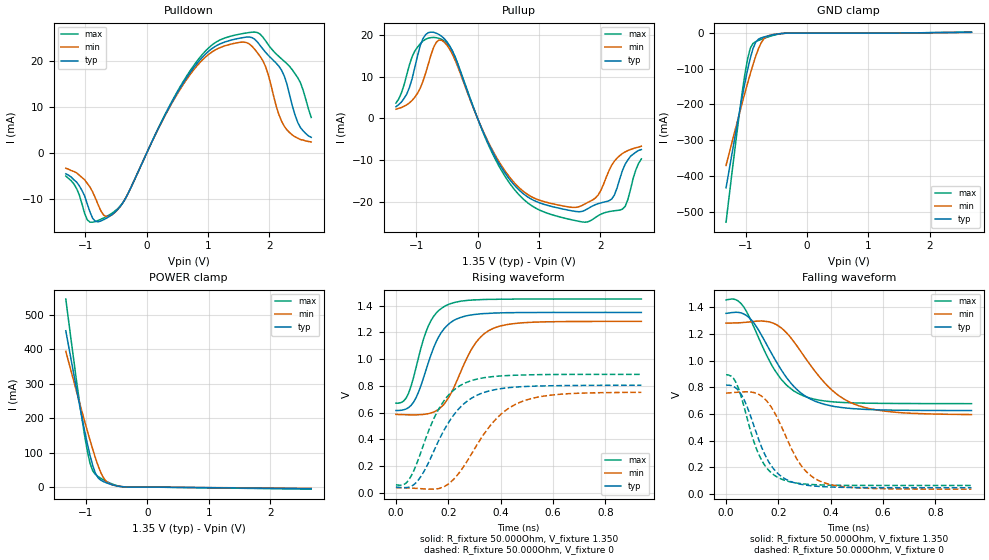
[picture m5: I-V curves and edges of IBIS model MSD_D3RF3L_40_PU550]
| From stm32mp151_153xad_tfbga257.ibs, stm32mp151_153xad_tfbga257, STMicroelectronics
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[Model] MSD_D3RF3L_40_PU550
Model_type   I/O
C_comp 2.425pF   2.340pF   2.550pF
Vinh = 810.000mV
Vinl = 540.000mV
Vmeas = 675.000mV
Vref = 675.000mV
[Model Spec]
Vinh   810.000mV   777.000mV   860.000mV
Vinl   540.000mV   507.000mV   590.000mV
Vmeas   675.000mV   642.000mV   725.000mV
Vref   675.000mV   642.000mV   725.000mV
[Temperature Range]   25.000   125.000   -40.000
[Voltage Range]   1.350V   1.283V   1.450V
[GND Clamp Reference]   0.00V   0.00V   0.00V
[Pulldown Reference]   0.00V   0.00V   0.00V
[POWER Clamp Reference]   1.350V   1.283V   1.450V
[Pullup Reference]   1.350V   1.283V   1.450V
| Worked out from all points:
|   slope of the pulldown table from 0 to 0.203 V, typ, clamps not added: 35.7 ohm
|   slope of the pullup table from 0 to 0.203 V, typ, clamps not added: 29.7 ohm
|   GND clamp passes 1 mA (typ) near -0.40 V on its own axis
|   POWER clamp passes 1 mA (typ) near -0.41 V on its own axis
|   rising waveform, R_fixture 50.000Ohm, V_fixture 1.350: 20-80 % time 86.8ps typ, 109ps min, 73.7ps max; typ from 0.615 V to 1.35 V
|   rising waveform, R_fixture 50.000Ohm, V_fixture 0: 20-80 % time 135ps typ, 161ps min, 116ps max; typ from 0.042 V to 0.804 V
|   falling waveform, R_fixture 50.000Ohm, V_fixture 1.350: 20-80 % time 147ps typ, 176ps min, 128ps max; typ from 1.35 V to 0.626 V
|   falling waveform, R_fixture 50.000Ohm, V_fixture 0: 20-80 % time 98.2ps typ, 116ps min, 84.8ps max; typ from 0.817 V to 0.048 V
[GND Clamp]
-1.318V   -433.6mA   -370.9mA   -529.9mA
-1.142V   -261.3mA   -253.2mA   -281mA
-1.055V   -178.7mA   -195.7mA   -165.9mA
-1.011V   -139.6mA   -167.6mA   -114.8mA
-966.7mV  -102.8mA   -140.1mA   -71.88mA
-922.7mV  -69.94mA   -113.6mA   -42.23mA
-878.8mV  -43.31mA   -88.24mA   -28.81mA
-790.9mV  -17.16mA   -44.13mA   -20.63mA
-703mV    -11.02mA   -16.16mA   -14.93mA
-527.3mV  -3.992mA   -3.373mA   -5.331mA
-307.6mV  -127.2uA   -185uA     -115.4uA
2.68V     2.404mA    2.042mA    2.844mA
[Power Clamp]
-1.33V    453mA      393.5mA    545mA
-1.111V   242.5mA    247.8mA    251.5mA
-1.023V   162.8mA    190.8mA    148.6mA
-978.8mV  125.6mA    162.8mA    104.1mA
-934.9mV  91.53mA    135.6mA    68.58mA
-890.9mV  62.14mA    109.2mA    46.94mA
-847mV    39.8mA     84.23mA    36.44mA
-803mV    26.44mA    61.41mA    30.34mA
-715.1mV  15.75mA    26.63mA    20.83mA
-671.2mV  12.52mA    16.53mA    16.67mA
-407.6mV  924.4uA    1.209mA    1.119mA
2.668V    -4.735mA   -3.8mA     -6.092mA
[Pulldown]
-1.318V   -4.5mA     -3.3mA     -5mA
-922.7mV  -12.81mA   -7.4mA     -14.98mA
-703mV    -14.45mA   -13.42mA   -14.07mA
-571.2mV  -13.38mA   -13.44mA   -13.08mA
-351.5mV  -9.986mA   -9.957mA   -9.952mA
747mV     18.14mA    17.69mA    18.58mA
1.098V    22.94mA    22.18mA    23.74mA
1.582V    25.02mA    24.02mA    25.91mA
1.889V    22.57mA    20.05mA    25.16mA
2.241V    16.68mA    5.8mA      19.86mA
2.461V    6.6mA      3.2mA      16.3mA
2.68V     3.4mA      2.4mA      7.7mA
[Pullup]
-1.33V    2.8mA      2.205mA    3.679mA
-1.155V   5.8mA      3.257mA    10.41mA
-978.8mV  15mA       6.025mA    17.12mA
-715.1mV  20.69mA    17.11mA    19.47mA
-451.5mV  17.37mA    16.56mA    17.25mA
251.5mV   -8.249mA   -7.87mA    -8.718mA
866.7mV   -19.34mA   -18.75mA   -20.84mA
1.702V    -22.37mA   -20.93mA   -24.89mA
1.965V    -20.5mA    -18.41mA   -23.39mA
2.185V    -19.39mA   -11.26mA   -22.3mA
2.361V    -12.5mA    -8.438mA   -21.81mA
2.668V    -7.5mA     -6.695mA   -9.748mA
[Ramp]
R_load=50.000Ohm
dV/dt_r   444.384mV/111.000ps  421.713mV/135.500ps  478.074mV/95.500ps
dV/dt_f   444.384mV/123.000ps  421.713mV/148.000ps  478.074mV/106.500ps
[Rising waveform]
R_fixture=50.000Ohm
V_fixture=1.350
V_fixture_min=1.283
V_fixture_max=1.450
0s        615.3mV    586.2mV    669.9mV
39ps      626.8mV    583.6mV    708.3mV
68ps      679.7mV    582.8mV    867.5mV
125ps     980.7mV    592.2mV    1.253V
163ps     1.166V     622.9mV    1.363V
202ps     1.263V     714mV      1.411V
298ps     1.334V     1.102V     1.444V
374ps     1.345V     1.232V     1.448V
527ps     1.349V     1.277V     1.45V
938ps     1.35V      1.283V     1.45V
[Rising waveform]
R_fixture=50.000Ohm
V_fixture=0
0s        42.3mV     37.23mV    59.07mV
39ps      37.84mV    35.64mV    71.73mV
87ps      98.19mV    31.03mV    256.5mV
135ps     268.7mV    26.28mV    511.2mV
173ps     427.7mV    36.75mV    657.3mV
269ps     680.2mV    226.3mV    825.4mV
384ps     773.5mV    554.9mV    871.7mV
480ps     793.8mV    681.4mV    881.1mV
623ps     801.6mV    736.4mV    885.3mV
938ps     804.4mV    751.5mV    886mV
[Falling waveform]
R_fixture=50.000Ohm
V_fixture=1.350
V_fixture_min=1.283
V_fixture_max=1.450
0s        1.355V     1.282V     1.455V
48ps      1.362V     1.284V     1.445V
96ps      1.307V     1.292V     1.298V
192ps     992.7mV    1.271V     912.4mV
230ps     876.4mV    1.211V     819.4mV
288ps     755.6mV    1.063V     743mV
403ps     661mV      782.2mV    692.5mV
508ps     637.8mV    661.5mV    682.7mV
652ps     628.9mV    612.9mV    679.4mV
938ps     626.1mV    596.2mV    678mV
[Falling waveform]
R_fixture=50.000Ohm
V_fixture=0
0s        816.8mV    757mV      894.4mV
29ps      806.6mV    761.3mV    866.4mV
48ps      775mV      764.4mV    790.6mV
77ps      672mV      767mV      594.8mV
125ps     407.8mV    747.7mV    297.7mV
163ps     242mV      679.4mV    178.6mV
211ps     133.1mV    509.5mV    113mV
288ps     72.88mV    211.4mV    78.26mV
374ps     55.47mV    85.15mV    68.07mV
938ps     47.64mV    37.02mV    64.63mV
